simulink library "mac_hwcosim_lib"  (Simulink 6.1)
undefined symbols (not defined in the file or in its folder): _hwcosim, JTAGRuntimeCosim, juan2, mac_clk_wrapper, netlist, XFix
libraries: XtremeDSPRunTimeCosim x1

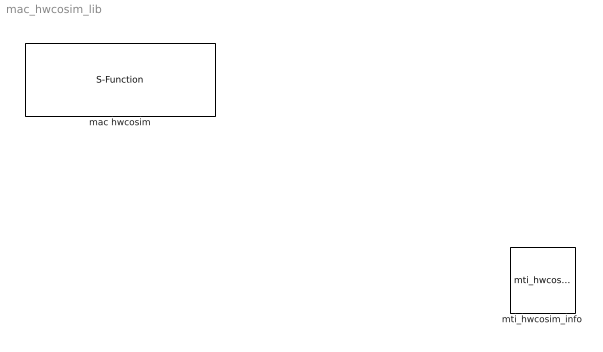
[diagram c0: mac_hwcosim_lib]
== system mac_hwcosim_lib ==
  mac hwcosim : S-Function  AncestorBlock=JTAGRuntimeCosim/_hwcosim  FunctionName=xlcosim  Parameters=sfcn_mwsv__  mask(Xilinx JTAG Hardware Co-Simulation){bitfileName=t:\juan2\netlist\mac_clk_wrapper.bit, clkSrc=Single Stepped, hasBufgmux=on, blkPeriod=0.5, IRLengths=[8,6], bscanPos=2, prtSignalType=XFix, prtNames={'gateway_in','gateway_in1','gateway_out'}, prtTypes={'Fix_8_6','Fix_8_6','Fix_16_12'}, prtDirs=[0,0,1], prtDataRates=[2,2,2]}
      mask prompts: bitfileName "Bit File Name"; clkSrc "Clock"; hasBufgmux "Supports BUFGMUX"; blkPeriod "Internal Block Period"; IRLengths "Instruction Reg Lengths"; bscanPos "BSCAN Position"; prtSignalType "Port Signal Type"; prtNames "Port Names (specified as cell array of strings)"; prtTypes "Port Types (specified as cell array of strings, eg 'Fix_8_7')"; prtDirs "Port Directions (specified as vector of integers, eg 'in'= 0 'out'=1)"; prtDataRates "Port Data Rates (specified as vector of integers)"
      mask help: Performs hardware co-simulation using JTAG and the Parallel Cable IV.
      mask init:
      | [bg,fg] = xlcmap('XBlock',1);
      | 
      | iPos = get_param(gcb,'Position');
      | iWidth=iPos(3)-iPos(1); iHeight=iPos(4)-iPos(2);
      | iCx=iWidth/2;
      | iCy=iHeight/2;
      | [logoX, logoY] = xlogo(iPos);
      | 
      | % support optional port that allows 
      | % selection between single-stepped and 
      | % free-running clocks during simulation
      | if (clkSrc == 3) 
      |   clkselprt = length(prtDirs)-sum(prtDirs)+1;
      |   clkseldir = 'input';
      |   clkselstr = 'clk_sel';
      | else
      |   clkselstr = '';
      |   if (length(prtDirs) == sum(prtDirs))
      |     clkseldir = 'output';
      |   else
      | 	clkseldir = 'input';
      |   end
      |   clkselprt = 1;
      | end
      | 
      | % assumes the cosim DLL resides in the same
      | % directory as the library containing the
      | % cosim block
      | libDir = which('JTAGRunTimeCosim');
      | binDir = fileparts(libDir);
      | 
      | % Extract target directory from bitstream
      | % name.
      | [targetDir,toplevelName] = fileparts(bitfileName);
      | 
      | % cosim DLL name goes here
      | engineDll = 'JTAGCosimEngine.dll';
      | 
      | % pass all mask workspace variables 
      | % to S-function
      | sfcn_mwsv__ = get_param(gcb, 'MaskWSVariables');
  mti_hwcosim_info : XtremeDSPRunTimeCosim/mti_hwcosim_info
